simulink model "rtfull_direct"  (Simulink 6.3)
settings: Solver=ode45  SolverMode=SingleTasking  StartTime=0.0  StopTime=inf  FixedStep=h  RelTol=1e-3  AbsTol=1e-6
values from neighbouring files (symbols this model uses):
  adingain = [1.2*(pi*2/620/3)*[1 -1 -1 1 1 1] 1]    [hwinit.m]
  adinoffs = [-421 -511 -568 -518 -521 -410    0]    [hwinit.m]
  daoutgain = 127*[1 -1 -1 1 1 1 1]    [hwinit.m]
  daoutoffs = 127*[1 1 1 1 0.98 1 0]    [hwinit.m]
  h = 0.01    [design_pol.m]    (also in design_rot.m; design_wrist.m; rtrobot_init.m = 0.05; simpleregret.m = cfg.h)
  joint = [1 2 3 4 5]    [design_pol.m]    (also in design_rot.m = [1 5]; design_wrist.m = [5]; rtrobot_init.m = joint(:)+(0:6:6*(n-1))')
  Kd = [0.4 0.1 0.1]    [design_pol.m]    (also in design_rot.m = [0.3 0.1]; design_wrist.m = 0.01; mc_approx_vectorized.m = cfg.Kd)
  Ki = [0.6 0.3 0.9]/3    [design_pol.m]    (also in design_rot.m = [0.1 0.1]; design_wrist.m = 0)
  Kp = [0.5 0.2 1.0]    [design_pol.m]    (also in design_rot.m = [0.4 2]; design_wrist.m = 1.5)
undefined symbols (not defined in the file or in its folder): COM1, L2, L3, No
libraries: xpclib x4, cstblocks x3, simulink x3, rtlib x1

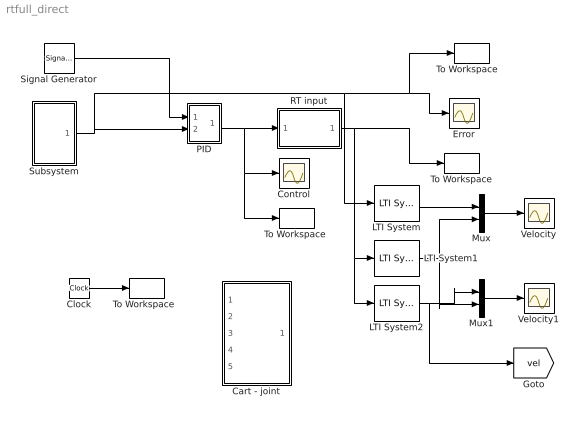
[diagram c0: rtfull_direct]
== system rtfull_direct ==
  Cart - joint : Subsystem
  Clock : Clock
  Control : Scope
  Error : Scope
  LTI System : cstblocks/LTI System  sys=Gder  IC=[]
  LTI System1 : cstblocks/LTI System  sys=Gder  IC=[]
  LTI System2 : cstblocks/LTI System  sys=Gder1  IC=[]
  Mux : Mux  Inputs=2
  Mux1 : Mux  Inputs=2
  PID : Subsystem
  RT input : Subsystem  InitFcn=rtclear all  mask{h=h, joint=joint, Port=COM1, laser=No, gripper=No}
      mask prompts: h "Sample time [s]:"; joint "Joints to control (e.g., [1 2 4])"; Port "Serial port:"; laser "Enable laser input"; gripper "Enable gripper current sensor"
      mask init:
      | hwinit;
      | sen = joint(:);                             % read joint angles
      | if strcmp(gripper,'Yes'),                   % if gripper current desired
      |     sen = [sen; 7];                         % add to the list
      | end;    
      |                                             
      | n = length(sen);                            % number of sensors to be read
      | sen = sen+(0:7:7*(n-1))';                   % convert into sequential index
      | sen_select = zeros(7,n);                    % prepare zeros
      | sen_select(sen) = 1;                        % assign 1 at the right places
      | 
      | act = joint(:);                             % control joint actuators
      | if strcmp(laser,'Yes'),                     % if laser desired
      |     act = [act; 7];                         % add to the list
      | end;    
      |                                             
      | n = length(act);                            % number of actuators to be controlled
      | act = act+(0:7:7*(n-1))';                   % convert into sequential index
      | act_select = zeros(7,n);                    % prepare zeros
      | act_select(act) = 1;                        % assign 1 at the right places
  Signal Generator : SignalGenerator  WaveForm=square  Amplitude=[0.4 0.3]  Frequency=1/5
  Subsystem : Subsystem
  To Workspace : ToWorkspace  VariableName=e  SampleTime=h  SaveFormat=Array
  "To Workspace " : ToWorkspace  VariableName=u  SampleTime=h  SaveFormat=Array
  "To Workspace  " : ToWorkspace  VariableName=t  SampleTime=h  SaveFormat=Array
  "To Workspace   " : ToWorkspace  VariableName=y  SampleTime=h  SaveFormat=Array
  Velocity : Scope
  Velocity1 : Scope
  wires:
  Subsystem/1(out_1) -> PID/2(in_2), "To Workspace   "/1, Error/1, LTI System/1
  RT input/1(Angles) -> To Workspace/1, LTI System2/1, LTI System1/1
  PID/1(out_1) -> Control/1, "To Workspace "/1, RT input/1(Motors)
  Clock/1 -> "To Workspace  "/1
  Signal Generator/1 -> PID/1(in_1)
  Mux/1 -> Velocity/1
  LTI System/1 -> Mux/1
  LTI System1/1 -> Mux/2, Mux1/2
  Mux1/1 -> Velocity1/1
  LTI System2/1 -> Mux1/1, [vel]

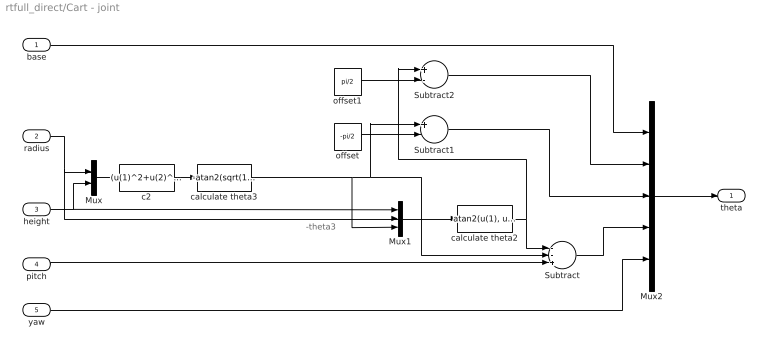
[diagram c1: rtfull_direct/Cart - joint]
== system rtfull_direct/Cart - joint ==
  note: -theta3
  base : Inport
  radius : Inport  Port=2
  height : Inport  Port=3
  pitch : Inport  Port=4
  yaw : Inport  Port=5
  Mux : Mux  Inputs=2
  Mux1 : Mux  Inputs=3
  Mux2 : Mux  Inputs=5
  Subtract : Sum  Inputs=--+  OutScaling=2^-10
  Subtract1 : Sum  Inputs=+-  OutScaling=2^-10
  Subtract2 : Sum  Inputs=+-  OutScaling=2^-10
  c2 : Fcn  Expr=(u(1)^2+u(2)^2-L2^2-L3^2)/(2*L2*L3)
  calculate theta2 : Fcn  Expr=atan2(u(1), u(2))-atan2(L3*sin(u(3)), L2+L3*cos(u(3)))
  calculate theta3 : Fcn  Expr=-atan2(sqrt(1-u(1)^2), u(1))
  offset : Constant  Value=-pi/2
  offset1 : Constant  Value=pi/2
  theta : Outport
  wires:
  height/1 -> Mux1/1, Mux/2
  Mux2/1 -> theta/1
  base/1 -> Mux2/1
  radius/1 -> Mux/1, Mux1/2
  c2/1 -> calculate theta3/1
  calculate theta3/1 -> Mux1/3, Subtract1/1, Subtract/2
  Mux/1 -> c2/1
  Mux1/1 -> calculate theta2/1
  calculate theta2/1 -> Subtract/1, Subtract2/1
  pitch/1 -> Subtract/3
  offset/1 -> Subtract1/2
  offset1/1 -> Subtract2/2
  Subtract1/1 -> Mux2/3
  Subtract2/1 -> Mux2/2
  Subtract/1 -> Mux2/4
  yaw/1 -> Mux2/5

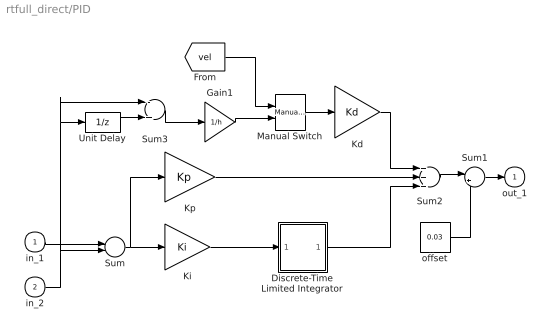
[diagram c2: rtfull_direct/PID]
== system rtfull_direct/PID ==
  in_1 : Inport
  in_2 : Inport  Port=2
  Discrete-Time Limited Integrator : Subsystem  mask(Discrete-Time Limited Integrator.){}
      mask help: Discrete-Time Limited Integrator.
      mask init:
      | lower_limit=@1;upper_limit=@2;X0=@3;Ts=@4;
  Gain1 : Gain  Gain=1/h  SampleTime=h
  Kd : Gain  Gain=Kd  SampleTime=h
  Ki : Gain  Gain=Ki  SampleTime=h
  Kp : Gain  Gain=Kp  SampleTime=h
  Manual Switch : simulink/Signal Routing/Manual Switch  sw=1  action=0
  Sum : Sum  Inputs=+-  SampleTime=h
  Sum1 : Sum  Inputs=|++
  Sum2 : Sum  Inputs=+++
  Sum3 : Sum  Inputs=-+  SampleTime=h
  Unit Delay : UnitDelay  SampleTime=h
  offset : Constant  Value=0.03
  out_1 : Outport  InitialOutput=0
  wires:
  Discrete-Time Limited Integrator/1(out_1) -> Sum2/3
  Ki/1 -> Discrete-Time Limited Integrator/1(in_1)
  Sum/1 -> Ki/1, Kp/1
  Kp/1 -> Sum2/2
  Kd/1 -> Sum2/1
  Unit Delay/1 -> Sum3/2
  in_1/1 -> Sum/1
  in_2/1 -> Sum/2, Unit Delay/1, Sum3/1
  Sum2/1 -> Sum1/1
  Sum1/1 -> out_1/1
  offset/1 -> Sum1/2
  Manual Switch/1 -> Kd/1
  Sum3/1 -> Gain1/1
  [vel] -> Manual Switch/1
  Gain1/1 -> Manual Switch/2

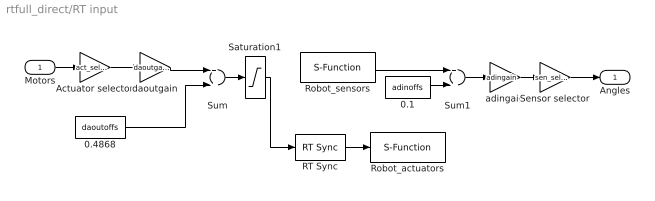
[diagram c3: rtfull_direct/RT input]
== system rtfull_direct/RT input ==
  Motors : Inport
  0.1 : Constant  Value=adinoffs
  0.4868 : Constant  Value=daoutoffs
  Actuator selector : Gain  Gain=act_select  Multiplication=Matrix(K*u)
  RT Sync : rtlib/RT Sync
  Robot_actuators : S-Function  FunctionName=sfserialout  Parameters=Ts, com  mask(Serial Out){Ts=h, Port=Port}
      mask prompts: Ts "Sample time:"; Port "Serial port:"
      mask help: Serial line output block
      mask init:
      | com = xserial('Port',Port,'Baudrate',115200);
  Robot_sensors : S-Function  FunctionName=sfserialin  Parameters=Ts, com  mask(Serial Out){Ts=h, Port=Port}
      mask prompts: Ts "Sample time:"; Port "Serial port:"
      mask help: Serial line output block
      mask init:
      | com = xserial('Port',Port,'Baudrate',115200);
  Saturation1 : Saturate  UpperLimit=255  LowerLimit=0
  Sensor selector : Gain  Gain=sen_select'  Multiplication=Matrix(K*u)
  Sum : Sum
  Sum1 : Sum
  adingain : Gain  Gain=adingain
  daoutgain : Gain  Gain=daoutgain
  Angles : Outport
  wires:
  RT Sync/1 -> Robot_actuators/1
  Actuator selector/1 -> daoutgain/1
  Sensor selector/1 -> Angles/1
  Saturation1/1 -> RT Sync/1
  daoutgain/1 -> Sum/1
  adingain/1 -> Sensor selector/1
  Robot_sensors/1 -> Sum1/1
  0.1/1 -> Sum1/2
  Sum1/1 -> adingain/1
  Motors/1 -> Actuator selector/1
  0.4868/1 -> Sum/2
  Sum/1 -> Saturation1/1

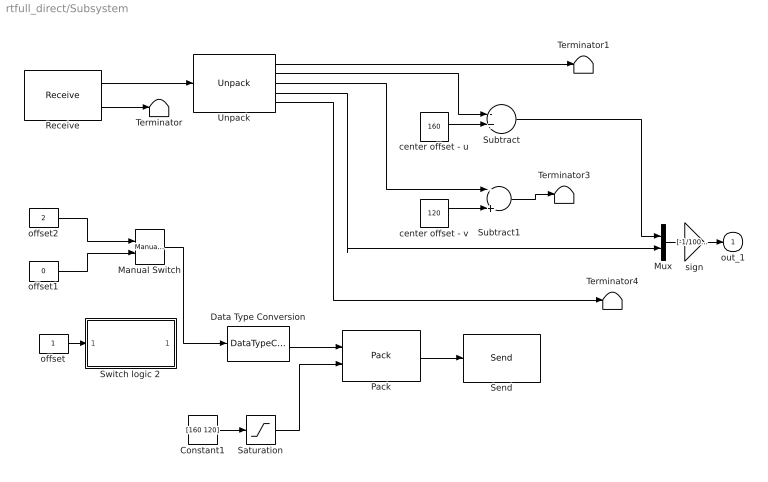
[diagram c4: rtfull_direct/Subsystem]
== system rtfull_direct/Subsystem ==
  Constant1 : Constant  Value=[160 120]
  Data Type Conversion : DataTypeConversion  OutDataTypeMode=uint8
  Manual Switch : simulink/Signal Routing/Manual Switch  sw=1  action=0
  Mux : Mux  Inputs=2
  Pack : xpclib/UDP/Pack  datatypes={'uint8','double'}  byteAlign=4
  Receive : xpclib/UDP/Receive  ipAddress=127.0.0.1  ipPort=6907  width=40  sampletime=h
  Saturation : Saturate  UpperLimit=[320 240]  LowerLimit=[0 0]
  Send : xpclib/UDP/Send  ipAddress=127.0.0.1  ipPort=6906  localPort=-1  sampletime=h
  Subtract : Sum  Inputs=-+  OutScaling=2^-10
  Subtract1 : Sum  Inputs=-+  OutScaling=2^-10
  Switch logic 2 : Subsystem
  Terminator{,1,3..4} (4 alike) : Terminator
  Unpack : xpclib/UDP/Unpack  dimensions={1,1,1,1,1}  datatypes={'double','double','double','double','double'}  byteAlign=4
  center offset - u : Constant  Value=160
  center offset - v : Constant  Value=120
  offset : Constant
  offset1 : Constant  Value=0
  offset2 : Constant  Value=2
  sign : Gain  Gain=[-1/100 -1]  SampleTime=h
  out_1 : Outport  InitialOutput=0
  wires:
  Receive/2 -> Terminator/1
  Receive/1 -> Unpack/1
  center offset - u/1 -> Subtract/2
  center offset - v/1 -> Subtract1/2
  Unpack/2 -> Subtract/1
  Unpack/3 -> Subtract1/1
  Unpack/4 -> Mux/2
  Subtract/1 -> Mux/1
  Unpack/5 -> Terminator4/1
  Pack/1 -> Send/1
  offset/1 -> Switch logic 2/1(In1)
  Constant1/1 -> Saturation/1
  Data Type Conversion/1 -> Pack/1
  Saturation/1 -> Pack/2
  Subtract1/1 -> Terminator3/1
  Manual Switch/1 -> Data Type Conversion/1
  offset2/1 -> Manual Switch/1
  offset1/1 -> Manual Switch/2
  Mux/1 -> sign/1
  Unpack/1 -> Terminator1/1
  sign/1 -> out_1/1

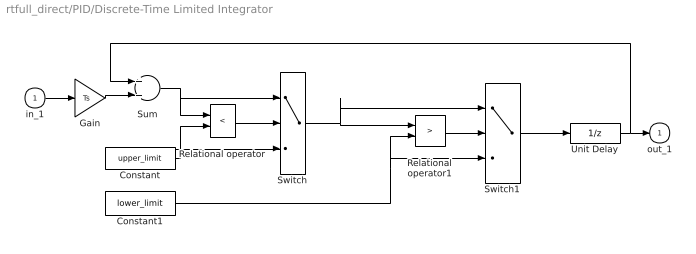
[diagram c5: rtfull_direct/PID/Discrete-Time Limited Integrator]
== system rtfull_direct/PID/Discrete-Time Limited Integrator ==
  in_1 : Inport
  Constant : Constant  Value=upper_limit
  Constant1 : Constant  Value=lower_limit
  Gain : Gain  Gain=Ts
  Relational operator : RelationalOperator  Operator=<
  Relational operator1 : RelationalOperator  Operator=>
  Sum : Sum
  Switch : Switch  Threshold=0.5
  Switch1 : Switch  Threshold=0.5
  Unit Delay : UnitDelay  X0=X0  SampleTime=Ts
  out_1 : Outport  InitialOutput=0
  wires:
  in_1/1 -> Gain/1
  Relational operator/1 -> Switch/2
  Sum/1 -> Relational operator/1, Switch/1
  Gain/1 -> Sum/2
  Constant/1 -> Relational operator/2, Switch/3
  Switch/1 -> Switch1/1, Relational operator1/1
  Relational operator1/1 -> Switch1/2
  Constant1/1 -> Switch1/3, Relational operator1/2
  Switch1/1 -> Unit Delay/1
  Unit Delay/1 -> Sum/1, out_1/1

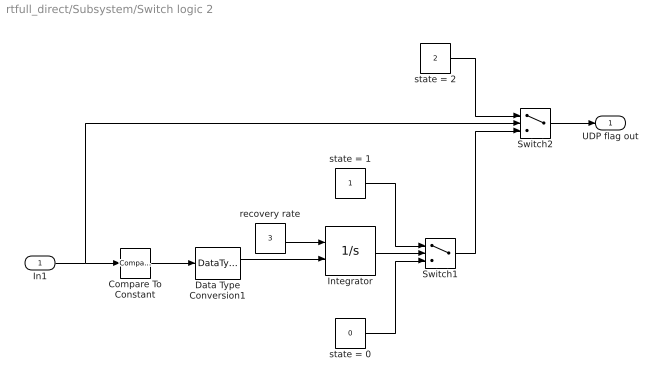
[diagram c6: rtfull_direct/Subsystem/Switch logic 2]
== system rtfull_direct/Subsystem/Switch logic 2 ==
  In1 : Inport
  Compare To Constant : simulink/Logic and Bit Operations/Compare To Constant  relop=<  const=1  LogicOutDataTypeMode=uint8  ZeroCross=off
  Data Type Conversion1 : DataTypeConversion  OutDataTypeMode=boolean
  Integrator : Integrator  ExternalReset=rising  LimitOutput=on  UpperSaturationLimit=1  LowerSaturationLimit=0
  Switch1 : Switch  Threshold=0.5
  Switch2 : Switch  Threshold=1
  recovery rate : Constant  Value=3
  state = 0 : Constant  Value=0
  state = 1 : Constant
  state = 2 : Constant  Value=2
  UDP flag out : Outport
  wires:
  state = 1/1 -> Switch1/1
  state = 0/1 -> Switch1/3
  Integrator/1 -> Switch1/2
  Data Type Conversion1/1 -> Integrator/2
  recovery rate/1 -> Integrator/1
  state = 2/1 -> Switch2/1
  Compare To Constant/1 -> Data Type Conversion1/1
  Switch1/1 -> Switch2/3
  Switch2/1 -> UDP flag out/1
  In1/1 -> Compare To Constant/1, Switch2/2
